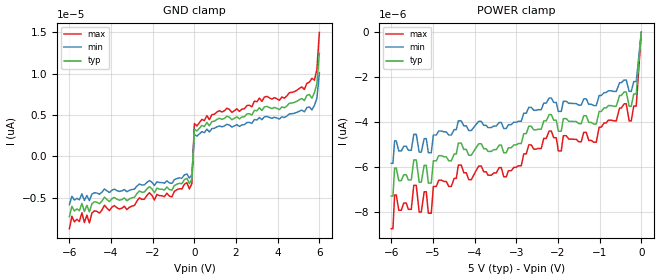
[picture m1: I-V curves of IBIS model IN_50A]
| TEXAS INSTRUMENTS INCORPORATED
| Standard Linear and Logic Group / High Volume Linear
| IBIS Model of TPD1E10B06-Q1
| Single Channel ESD Protection Device
| This file contains package information for the following:
|  QFN 2-pin (DPY) package as [Component] TPD1E10B06-Q1_DPY
| This device can be powered at the following Vccs:
|  5 volt Vcc
| This file provides unique models under the [Model Selector] for each Vcc.
| For operation at a specific Vcc, select the appropriate model after each
| [Model Selector] keyword.
[IBIS Ver]   3.2
[Comment char]  |_char
[File Name]   tpd1e10b06-q1.ibs
[File Rev]   0 | A1
[Date]   ??????
[Source]   Data created from TI-SPICE simulations at TI-SLL/HVL.
   The following is an IBIS list for the TPD1E10B06-Q1.
   Please contact sllibis@ti.com with questions and
   comments concerning SLL IBIS models.
[Notes]   Revision_History:
[Disclaimer]
| This model is designed as an aid for customers of Texas Instruments.
| TI and its licensors and suppliers make no warranties, either expressed
| or implied, with respect to this  model, including the warranties of
| merchantability or fitness for a particular purpose. The model is
| provided solely on an "as is" basis. The entire risk as to its quality
| and performance is with the customer.
[Copyright]
| (C) Copyright 2016 Texas Instruments Incorporated. All rights reserved.
| Component TPD1E10B06-Q1_DPY 2-PIN QFN
[Component]   TPD1E10B06-Q1_DPY
[Manufacturer]   Texas Instruments, Inc.
[Package]
|   typ   min   max
R_pkg   6.000e-02   5.900e-02   6.100e-02
L_pkg   5.003e-10   4.430e-10   5.015e-10
C_pkg   2.000e-14   1.990e-14   2.010e-14
[Pin]   signal_name   model_name   R_pin   L_pin   C_pin
1   1   IN_50A   6.100e-02   4.430e-10   1.990e-14
2   2   GND   6.100e-02   4.430e-10   1.990e-14
| Models and submodels in the file (1): IN_50A (Input)
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| Model IN
[Model]   IN_50A
Model_type  Input
Vinl=0
Vinh=5
| variable   typ   min   max
C_comp   12.4pF   11.4pF   13.4pF
[Temperature Range]   40   100   -40
| Ambient temperature   25   85   -40
[Voltage range]   5   5   5
[GND Clamp]
| IN_50A
|   Voltage   I(typ)   I(min)   I(max)
-6V       -7.29pA    -5.83pA    -8.74pA
-5.88V    -6.04pA    -4.83pA    -7.24pA
-5.04V    -6.71pA    -5.36pA    -8.05pA
-4.32V    -4.93pA    -3.94pA    -5.91pA
-3.24V    -5.36pA    -4.28pA    -6.43pA
-240mV    -3.29pA    -2.63pA    -3.94pA
-120mV    -2.74pA    -2.19pA    -3.28pA
0V        3.32pA     2.65pA     3.98pA
5.28V     6.75pA     5.4pA      8.1pA
5.76V     7.69pA     6.15pA     9.22pA
5.88V     8.8pA      7.04pA     10.5pA
6V        12.5pA     10.1pA     15pA
[POWER Clamp]
| IN_50A
|   Voltage   I(typ)   I(min)   I(max)
-6V       -7.29pA    -5.83pA    -8.74pA
-5.92V    -6.04pA    -4.83pA    -7.24pA
-5.4V     -5.68pA    -4.54pA    -6.81pA
-5.04V    -6.71pA    -5.36pA    -8.05pA
-4.99V    -5.72pA    -4.57pA    -6.86pA
-4.39V    -4.93pA    -3.94pA    -5.91pA
-3.24V    -5.36pA    -4.28pA    -6.43pA
-2.21V    -3.66pA    -2.92pA    -4.39pA
-1.92V    -4.4pA     -3.52pA    -5.28pA
-240mV    -3.29pA    -2.63pA    -3.94pA
-120mV    -2.74pA    -2.19pA    -3.28pA
0V        0A         0A         0A
